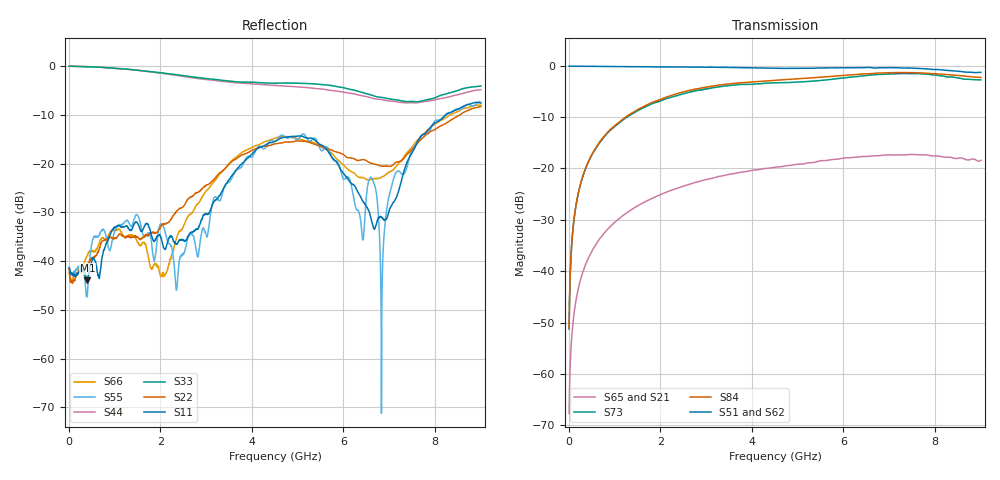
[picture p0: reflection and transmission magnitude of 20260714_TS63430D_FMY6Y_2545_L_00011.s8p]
# GHz S DB R 50
! CMT, SN0916, 25263762, 26.7.0
! Date: 15.07.2026 14:52:55
! Data: Format
! Freq S1.1:dB/Ang S1.2:dB/Ang S1.3:dB/Ang S1.4:dB/Ang S1.5:dB/Ang S1.6:dB/Ang S1.7:dB/Ang S1.8:dB/Ang
!  S2.1:dB/Ang S2.2:dB/Ang S2.3:dB/Ang S2.4:dB/Ang S2.5:dB/Ang S2.6:dB/Ang S2.7:dB/Ang S2.8:dB/Ang
!  S3.1:dB/Ang S3.2:dB/Ang S3.3:dB/Ang S3.4:dB/Ang S3.5:dB/Ang S3.6:dB/Ang S3.7:dB/Ang S3.8:dB/Ang
!  S4.1:dB/Ang S4.2:dB/Ang S4.3:dB/Ang S4.4:dB/Ang S4.5:dB/Ang S4.6:dB/Ang S4.7:dB/Ang S4.8:dB/Ang
!  S5.1:dB/Ang S5.2:dB/Ang S5.3:dB/Ang S5.4:dB/Ang S5.5:dB/Ang S5.6:dB/Ang S5.7:dB/Ang S5.8:dB/Ang
!  S6.1:dB/Ang S6.2:dB/Ang S6.3:dB/Ang S6.4:dB/Ang S6.5:dB/Ang S6.6:dB/Ang S6.7:dB/Ang S6.8:dB/Ang
!  S7.1:dB/Ang S7.2:dB/Ang S7.3:dB/Ang S7.4:dB/Ang S7.5:dB/Ang S7.6:dB/Ang S7.7:dB/Ang S7.8:dB/Ang
!  S8.1:dB/Ang S8.2:dB/Ang S8.3:dB/Ang S8.4:dB/Ang S8.5:dB/Ang S8.6:dB/Ang S8.7:dB/Ang S8.8:dB/Ang
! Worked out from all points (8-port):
!   2001 points, 10 MHz to 9 GHz, reference 50 ohm
!   strongest paths, dB at 10 MHz, 2.257 GHz, 4.505 GHz, 6.753 GHz, 9 GHz:
!     S51: -0.1, -0.2, -0.5, -0.4, -1.3
!     S62: -0.1, -0.3, -0.5, -0.4, -1.2
!     S84: -51.1, -5.8, -2.8, -1.4, -2.3
!     S73: -51.3, -6.1, -3.3, -1.7, -2.8
!     S65: -67.7, -24.2, -19.8, -17.5, -18.4
!     S21: -67.6, -24.2, -19.8, -17.5, -18.4
!   lowest |S11| = -44.0 dB at 410.1 MHz (marker M1), VSWR 1.01, Z = 50.3 - j0.579 ohm
!   |S11| at or under -10 dB: start of sweep to 8.236 GHz
